FUNCTION FC 53 : VOID
TITLE =
VERSION : 0.1


VAR_INPUT
  Continuity_Enabled : BOOL ;
  Start : BOOL ;
END_VAR
VAR_OUTPUT
  HV_Contactor : BOOL ;
  Cell1_Contactor : BOOL ;
  Cell2_Contactor : BOOL ;
  Cell3_Contactor : BOOL ;
  Cell4_Contactor : BOOL ;
  Cell5_Contactor : BOOL ;
  Cell6_Contactor : BOOL ;
  Start_measure : BOOL ;
  Bypass_Contactor : BOOL ;
  Short_Circuit_Fail : BOOL ;
  Continuity_Fail : BOOL ;
  Test_Completed : BOOL ;
END_VAR
VAR_TEMP
  Actual_time : INT ;
  remaining_time : INT ;
END_VAR
BEGIN
NETWORK
TITLE =
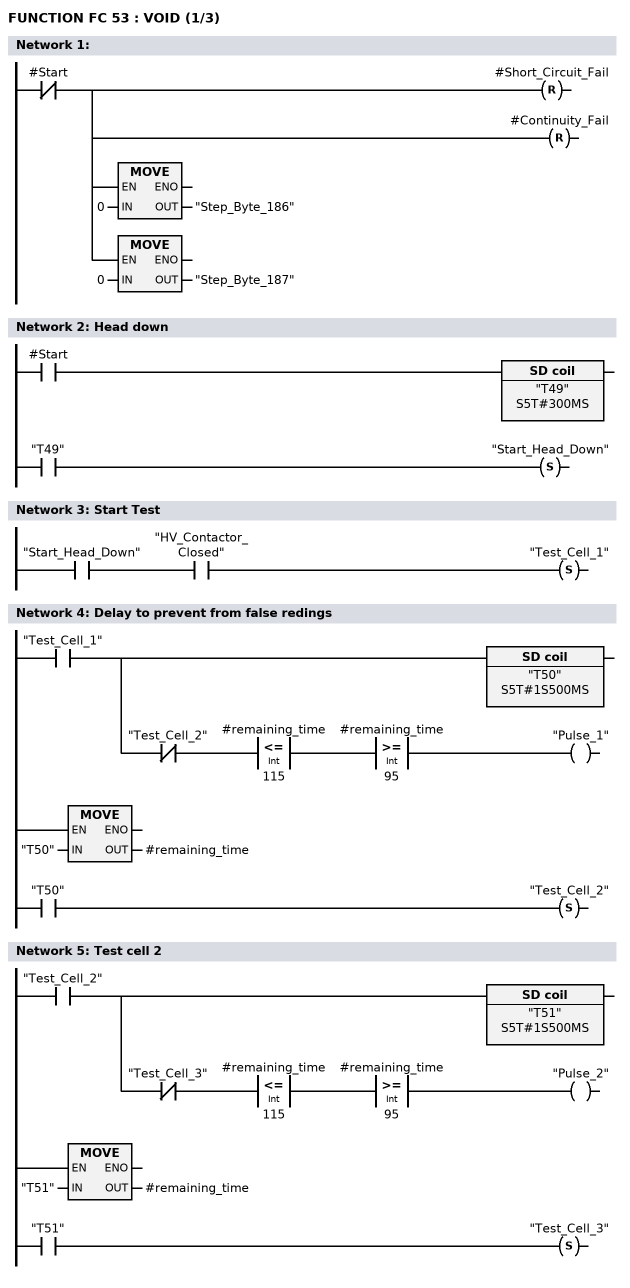
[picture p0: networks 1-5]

      UN    #Start;
      =     L      4.0;
      U     L      4.0;
      BLD   102;
      R     #Short_Circuit_Fail;
      U     L      4.0;
      BLD   102;
      R     #Continuity_Fail;
      U     L      4.0;
      SPBNB _001;
      L     0;
      T     "Step_Byte_186";
_001: NOP   0;
      U     L      4.0;
      SPBNB _002;
      L     0;
      T     "Step_Byte_187";
_002: NOP   0;
NETWORK
TITLE =Head down



      U     #Start;
      L     S5T#300MS;
      SE    "T49";
      NOP   0;
      NOP   0;
      NOP   0;
      U     "T49";
      S     "Start_Head_Down";
NETWORK
TITLE =Start Test

      U     "Start_Head_Down";
      U     "HV_Contactor_Closed";
      S     "Test_Cell_1";
NETWORK
TITLE =Delay to prevent from false redings

      U     "Test_Cell_1";
      =     L      4.0;
      U     L      4.0;
      L     S5T#1S500MS;
      SE    "T50";
      NOP   0;
      L     "T50";
      T     #remaining_time;
      NOP   0;
      U     "T50";
      S     "Test_Cell_2";
      U     L      4.0;
      UN    "Test_Cell_2";
      U(    ;
      L     #remaining_time;
      L     115;
      <=I   ;
      )     ;
      U(    ;
      L     #remaining_time;
      L     95;
      >=I   ;
      )     ;
      =     "Pulse_1";
NETWORK
TITLE =Test cell 2

      U     "Test_Cell_2";
      =     L      4.0;
      U     L      4.0;
      L     S5T#1S500MS;
      SE    "T51";
      NOP   0;
      L     "T51";
      T     #remaining_time;
      NOP   0;
      U     "T51";
      S     "Test_Cell_3";
      U     L      4.0;
      UN    "Test_Cell_3";
      U(    ;
      L     #remaining_time;
      L     115;
      <=I   ;
      )     ;
      U(    ;
      L     #remaining_time;
      L     95;
      >=I   ;
      )     ;
      =     "Pulse_2";
NETWORK
TITLE =Controllo Orientamento Coperchio (Coperchio in Posizione Errata)
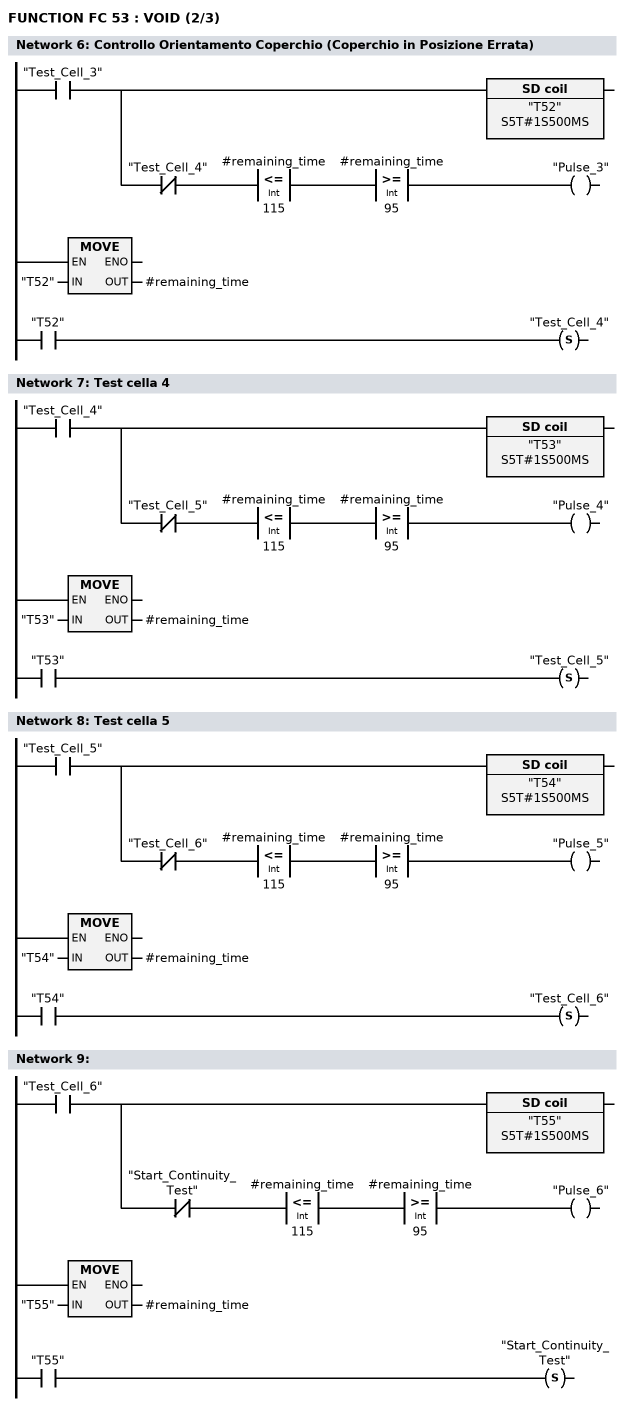
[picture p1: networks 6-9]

      U     "Test_Cell_3";
      =     L      4.0;
      U     L      4.0;
      L     S5T#1S500MS;
      SE    "T52";
      NOP   0;
      L     "T52";
      T     #remaining_time;
      NOP   0;
      U     "T52";
      S     "Test_Cell_4";
      U     L      4.0;
      UN    "Test_Cell_4";
      U(    ;
      L     #remaining_time;
      L     115;
      <=I   ;
      )     ;
      U(    ;
      L     #remaining_time;
      L     95;
      >=I   ;
      )     ;
      =     "Pulse_3";
NETWORK
TITLE =Test cella 4

      U     "Test_Cell_4";
      =     L      4.0;
      U     L      4.0;
      L     S5T#1S500MS;
      SE    "T53";
      NOP   0;
      L     "T53";
      T     #remaining_time;
      NOP   0;
      U     "T53";
      S     "Test_Cell_5";
      U     L      4.0;
      UN    "Test_Cell_5";
      U(    ;
      L     #remaining_time;
      L     115;
      <=I   ;
      )     ;
      U(    ;
      L     #remaining_time;
      L     95;
      >=I   ;
      )     ;
      =     "Pulse_4";
NETWORK
TITLE =Test cella 5

      U     "Test_Cell_5";
      =     L      4.0;
      U     L      4.0;
      L     S5T#1S500MS;
      SE    "T54";
      NOP   0;
      L     "T54";
      T     #remaining_time;
      NOP   0;
      U     "T54";
      S     "Test_Cell_6";
      U     L      4.0;
      UN    "Test_Cell_6";
      U(    ;
      L     #remaining_time;
      L     115;
      <=I   ;
      )     ;
      U(    ;
      L     #remaining_time;
      L     95;
      >=I   ;
      )     ;
      =     "Pulse_5";
NETWORK
TITLE =

      U     "Test_Cell_6";
      =     L      4.0;
      U     L      4.0;
      L     S5T#1S500MS;
      SE    "T55";
      NOP   0;
      L     "T55";
      T     #remaining_time;
      NOP   0;
      U     "T55";
      S     "Start_Continuity_Test";
      U     L      4.0;
      UN    "Start_Continuity_Test";
      U(    ;
      L     #remaining_time;
      L     115;
      <=I   ;
      )     ;
      U(    ;
      L     #remaining_time;
      L     95;
      >=I   ;
      )     ;
      =     "Pulse_6";
NETWORK
TITLE =Attivazione dei contattori di bypass
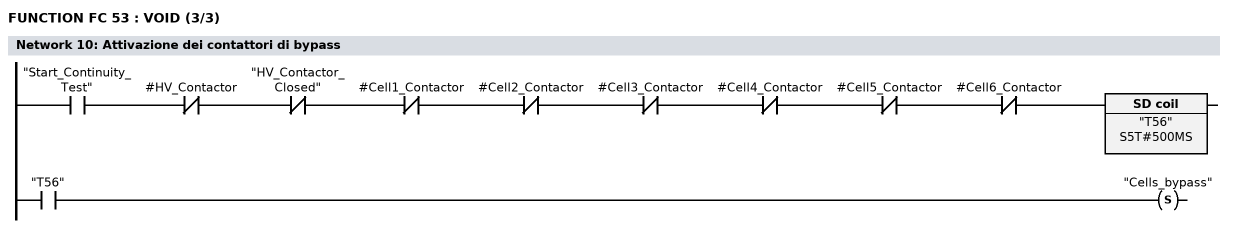
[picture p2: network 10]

      U     "Start_Continuity_Test";
      UN    #HV_Contactor;
      UN    "HV_Contactor_Closed";
      UN    #Cell1_Contactor;
      UN    #Cell2_Contactor;
      UN    #Cell3_Contactor;
      UN    #Cell4_Contactor;
      UN    #Cell5_Contactor;
      UN    #Cell6_Contactor;
      L     S5T#500MS;
      SE    "T56";
      NOP   0;
      NOP   0;
      NOP   0;
      U     "T56";
      S     "Cells_bypass";
NETWORK
TITLE =Verifica esito della continuità

      U(    ;
      U     "Cells_bypass";
      L     S5T#1S500MS;
      SE    "T57";
      NOP   0;
      NOP   0;
      NOP   0;
      U     "T57";
      )     ;
      UN    "Test_Completed";
      =     L      4.0;
      U     L      4.0;
      U     #Continuity_Enabled;
      UN    "Continuity_signal";
      S     #Continuity_Fail;
      U     L      4.0;
      UN    #Continuity_Enabled;
      R     #Continuity_Fail;
      U     L      4.0;
      BLD   102;
      S     "Test_Completed";
NETWORK
TITLE =
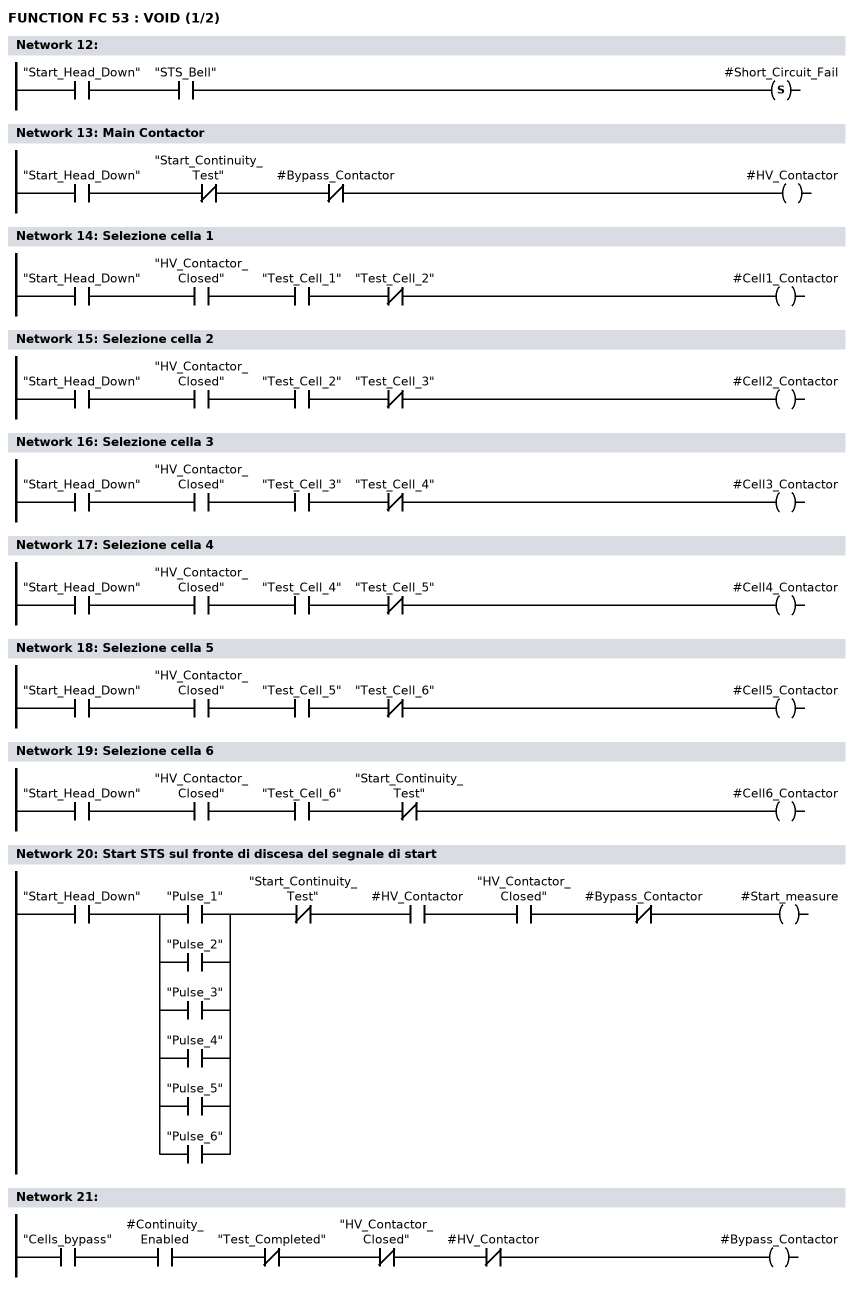
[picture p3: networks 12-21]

      U     "Start_Head_Down";
      U     "STS_Bell";
      S     #Short_Circuit_Fail;
NETWORK
TITLE =Main Contactor

      U     "Start_Head_Down";
      UN    "Start_Continuity_Test";
      UN    #Bypass_Contactor;
      =     #HV_Contactor;
NETWORK
TITLE =Selezione cella 1

      U     "Start_Head_Down";
      U     "HV_Contactor_Closed";
      U     "Test_Cell_1";
      UN    "Test_Cell_2";
      =     #Cell1_Contactor;
NETWORK
TITLE =Selezione cella 2

      U     "Start_Head_Down";
      U     "HV_Contactor_Closed";
      U     "Test_Cell_2";
      UN    "Test_Cell_3";
      =     #Cell2_Contactor;
NETWORK
TITLE =Selezione cella 3

      U     "Start_Head_Down";
      U     "HV_Contactor_Closed";
      U     "Test_Cell_3";
      UN    "Test_Cell_4";
      =     #Cell3_Contactor;
NETWORK
TITLE =Selezione cella 4

      U     "Start_Head_Down";
      U     "HV_Contactor_Closed";
      U     "Test_Cell_4";
      UN    "Test_Cell_5";
      =     #Cell4_Contactor;
NETWORK
TITLE =Selezione cella 5

      U     "Start_Head_Down";
      U     "HV_Contactor_Closed";
      U     "Test_Cell_5";
      UN    "Test_Cell_6";
      =     #Cell5_Contactor;
NETWORK
TITLE =Selezione cella 6

      U     "Start_Head_Down";
      U     "HV_Contactor_Closed";
      U     "Test_Cell_6";
      UN    "Start_Continuity_Test";
      =     #Cell6_Contactor;
NETWORK
TITLE =Start STS sul fronte di discesa del segnale di start

      U     "Start_Head_Down";
      U(    ;
      O     "Pulse_1";
      O     "Pulse_2";
      O     "Pulse_3";
      O     "Pulse_4";
      O     "Pulse_5";
      O     "Pulse_6";
      )     ;
      UN    "Start_Continuity_Test";
      U     #HV_Contactor;
      U     "HV_Contactor_Closed";
      UN    #Bypass_Contactor;
      =     #Start_measure;
NETWORK
TITLE =

      U     "Cells_bypass";
      U     #Continuity_Enabled;
      UN    "Test_Completed";
      UN    "HV_Contactor_Closed";
      UN    #HV_Contactor;
      =     #Bypass_Contactor;
NETWORK
TITLE =Fine ciclo di test
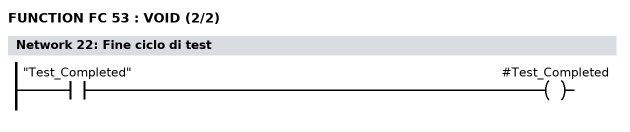
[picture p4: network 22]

      U     "Test_Completed";
      =     #Test_Completed;
END_FUNCTION

